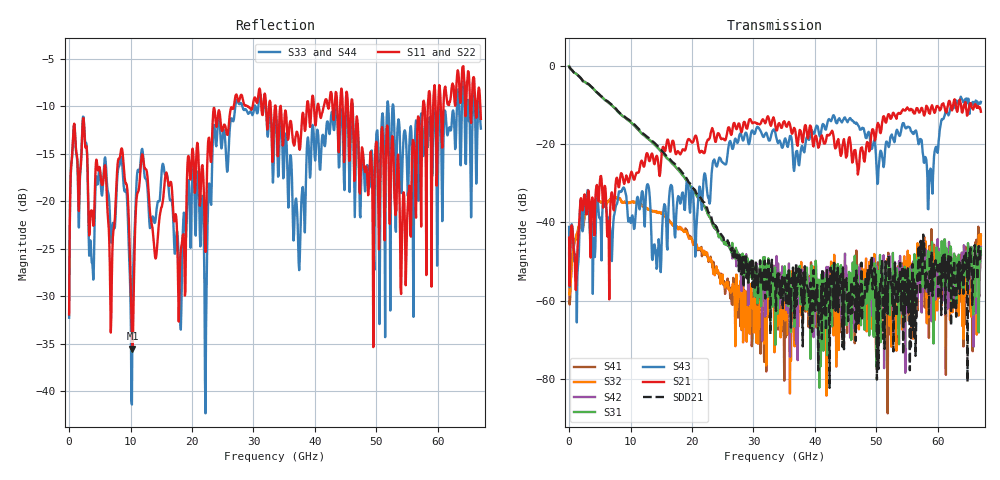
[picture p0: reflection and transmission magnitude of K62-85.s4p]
!Agilent Technologies,N5247A,US50470101,A.10.25.02
!Agilent N5247A: A.10.25.02
!Date: Tuesday, May 12, 2015 13:45:49
!Correction: Sdd11(Full 4 Port(1,2,3,4))
!Sdc11(Full 4 Port(1,2,3,4))
!Sdd12(Full 4 Port(1,2,3,4))
!Sdc12(Full 4 Port(1,2,3,4))
!Scd11(Full 4 Port(1,2,3,4))
!Scc11(Full 4 Port(1,2,3,4))
!Scd12(Full 4 Port(1,2,3,4))
!Scc12(Full 4 Port(1,2,3,4))
!Sdd21(Full 4 Port(1,2,3,4))
!Sdc21(Full 4 Port(1,2,3,4))
!Sdd22(Full 4 Port(1,2,3,4))
!Sdc22(Full 4 Port(1,2,3,4))
!Scd21(Full 4 Port(1,2,3,4))
!Scc21(Full 4 Port(1,2,3,4))
!Scd22(Full 4 Port(1,2,3,4))
!Scc22(Full 4 Port(1,2,3,4))
!Balanced Topology: BBAL
!S4P File: Measurements: <Sdd11,Sdc11,Sdd12,Sdc12>,
!<Scd11,Scc11,Scd12,Scc12>,
!<Sdd21,Sdc21,Sdd22,Sdc22>,
!<Scd21,Scc21,Scd22,Scc22>:
# Hz S  dB  R 50
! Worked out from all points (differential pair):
!   801 points, 10 MHz to 67 GHz, reference 50 ohm
!   strongest paths, dB at 10 MHz, 16.76 GHz, 33.51 GHz, 50.25 GHz, 67 GHz:
!     S21: -43.9, -19.5, -14.8, -14.6, -11.7
!     S43: -41.2, -30.9, -16.8, -29.9, -9.2
!     S31: -0.1, -24.9, -51.5, -61.8, -48.2
!     S42: -0.1, -24.9, -52.5, -56.8, -46.2
!     S32: -46.7, -40.4, -66.7, -57.2, -43.0
!     S41: -47.9, -40.5, -57.0, -50.2, -43.6
!   taken as a pair (ports 1,2 in; 3,4 out), SDD21 dB: -0.1, -24.5, -54.0, -58.5, -46.8
!   lowest |S11| = -35.5 dB at 10.31 GHz (marker M1), VSWR 1.03, Z = 51.7 + j0.0469 ohm
!   |S11| at or under -10 dB: start of sweep to 26.81 GHz; 34.43 GHz to 38.69 GHz (4.258 GHz wide, 11.6 % of centre); 46.13 GHz to 57.58 GHz (11.44 GHz wide, 22.1 % of centre)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
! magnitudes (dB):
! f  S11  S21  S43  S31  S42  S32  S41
! 10 MHz  -31.9  -43.9  -41.2  -0.1  -0.1  -46.7  -47.9
! 8.467 GHz  -14.5  -27.4  -32.1  -12.5  -12.5  -34.5  -34.4
! 10.31 GHz  -35.5  -27.6  -38.2  -14.8  -14.8  -34.8  -34.7
! 11.73 GHz  -15.7  -24.3  -33.5  -17.2  -17.2  -35.4  -35.4
! 31.24 GHz  -9.5  -14.5  -16.9  -61.4  -58.9  -57.2  -53.6
! 58.71 GHz  -8.8  -12.2  -27.5  -53.7  -52.3  -46.2  -48.2
! 67 GHz  -11.3  -11.7  -9.2  -48.2  -46.2  -43.0  -43.6
